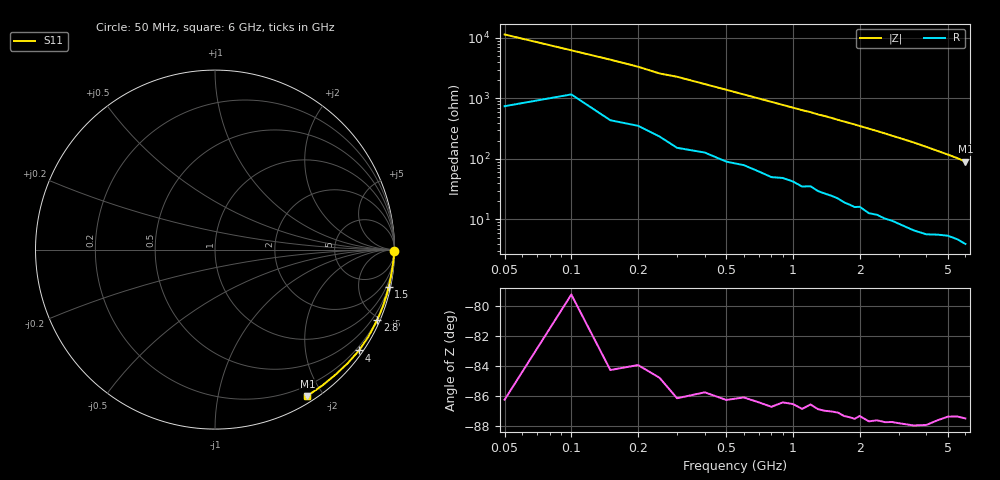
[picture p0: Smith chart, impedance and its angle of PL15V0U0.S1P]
! Infineon Technologies  Discrete & RF Semiconductors
! BAR 64-04W /-05W /-06W
! Si PIN Diode in SOT323
! VR = 15 V
! S-Parameters:  October  2008
# GHz  S  MA  R  50
!  f  S11
! GHz  MAG  ANG
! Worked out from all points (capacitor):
!   34 points, 50 MHz to 6 GHz, reference 50 ohm
!   read as one part to ground: C = 259 fF near 50 MHz
!   lowest |Z| = 90.7 ohm at 6 GHz (marker M1)
!   S11 on the Smith chart (normalised r, x): 50 MHz: open; 1.5 GHz: 0.49, -9.49; 2.8 GHz: 0.19, -4.84; 4 GHz: 0.11, -3.17; 6 GHz: 0.08, -1.81
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0.05  0.9994 -0.5
0.1  0.997 -0.9
0.15  0.9977 -1.3
0.2  0.9969 -1.7
0.25  0.9965 -2.2
0.3  0.9971 -2.5
0.8  0.9936 -6.5
0.9  0.9921 -7.3
1.1  0.9916 -8.9
1.2  0.9901 -9.6
1.3  0.9902 -10.5
1.4  0.9899 -11.2
1.5  0.9893 -12.0
1.6  0.9889 -12.9
1.7  0.9891 -13.7
1.9  0.9887 -15.3
2  0.9872 -16.2
2.2  0.9878 -17.9
2.4  0.9863 -19.6
2.6  0.9858 -21.4
2.8  0.9846 -23.3
3  0.984 -25.1
3.5  0.9826 -29.8
4  0.9797 -35.0
4.5  0.9736 -40.4
5  0.9679 -45.8
5.5  0.9648 -51.5
6  0.9639 -57.7
